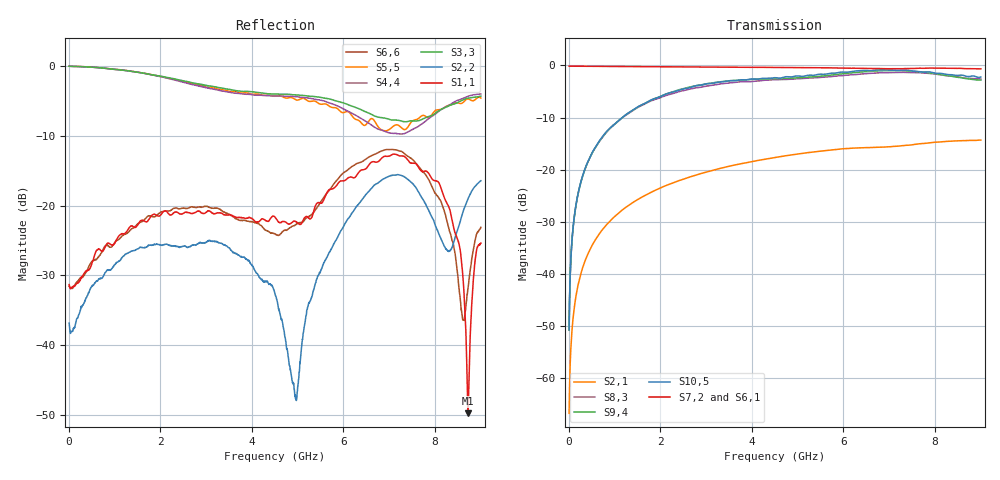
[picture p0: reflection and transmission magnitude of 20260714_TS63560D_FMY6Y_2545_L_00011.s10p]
# GHz S DB R 50
! CMT, SN0916, 25263762, 26.7.0
! Date: 15.07.2026 13:32:48
! Data: Format
! Freq S1.1:dB/Ang S1.2:dB/Ang S1.3:dB/Ang S1.4:dB/Ang S1.5:dB/Ang S1.6:dB/Ang S1.7:dB/Ang S1.8:dB/Ang S1.9:dB/Ang S1.10:dB/Ang
!  S2.1:dB/Ang S2.2:dB/Ang S2.3:dB/Ang S2.4:dB/Ang S2.5:dB/Ang S2.6:dB/Ang S2.7:dB/Ang S2.8:dB/Ang S2.9:dB/Ang S2.10:dB/Ang
!  S3.1:dB/Ang S3.2:dB/Ang S3.3:dB/Ang S3.4:dB/Ang S3.5:dB/Ang S3.6:dB/Ang S3.7:dB/Ang S3.8:dB/Ang S3.9:dB/Ang S3.10:dB/Ang
!  S4.1:dB/Ang S4.2:dB/Ang S4.3:dB/Ang S4.4:dB/Ang S4.5:dB/Ang S4.6:dB/Ang S4.7:dB/Ang S4.8:dB/Ang S4.9:dB/Ang S4.10:dB/Ang
!  S5.1:dB/Ang S5.2:dB/Ang S5.3:dB/Ang S5.4:dB/Ang S5.5:dB/Ang S5.6:dB/Ang S5.7:dB/Ang S5.8:dB/Ang S5.9:dB/Ang S5.10:dB/Ang
!  S6.1:dB/Ang S6.2:dB/Ang S6.3:dB/Ang S6.4:dB/Ang S6.5:dB/Ang S6.6:dB/Ang S6.7:dB/Ang S6.8:dB/Ang S6.9:dB/Ang S6.10:dB/Ang
!  S7.1:dB/Ang S7.2:dB/Ang S7.3:dB/Ang S7.4:dB/Ang S7.5:dB/Ang S7.6:dB/Ang S7.7:dB/Ang S7.8:dB/Ang S7.9:dB/Ang S7.10:dB/Ang
!  S8.1:dB/Ang S8.2:dB/Ang S8.3:dB/Ang S8.4:dB/Ang S8.5:dB/Ang S8.6:dB/Ang S8.7:dB/Ang S8.8:dB/Ang S8.9:dB/Ang S8.10:dB/Ang
!  S9.1:dB/Ang S9.2:dB/Ang S9.3:dB/Ang S9.4:dB/Ang S9.5:dB/Ang S9.6:dB/Ang S9.7:dB/Ang S9.8:dB/Ang S9.9:dB/Ang S9.10:dB/Ang
!  S10.1:dB/Ang S10.2:dB/Ang S10.3:dB/Ang S10.4:dB/Ang S10.5:dB/Ang S10.6:dB/Ang S10.7:dB/Ang S10.8:dB/Ang S10.9:dB/Ang S10.10:dB/Ang
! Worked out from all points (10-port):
!   2001 points, 10 MHz to 9 GHz, reference 50 ohm
!   strongest paths, dB at 10 MHz, 2.257 GHz, 4.505 GHz, 6.753 GHz, 9 GHz:
!     S7,2: -0.1, -0.3, -0.4, -0.6, -0.6
!     S6,1: -0.2, -0.4, -0.5, -0.7, -0.6
!     S10,5: -50.8, -5.1, -2.3, -0.8, -2.2
!     S9,4: -50.9, -5.1, -2.5, -1.0, -2.8
!     S8,3: -50.7, -5.4, -2.7, -1.4, -2.6
!     S2,1: -66.8, -22.6, -17.7, -15.7, -14.3
!   lowest |S11| = -49.7 dB at 8.721 GHz (marker M1), VSWR 1.01, Z = 49.9 + j0.297 ohm
!   |S11| at or under -10 dB: start of sweep to end of sweep
